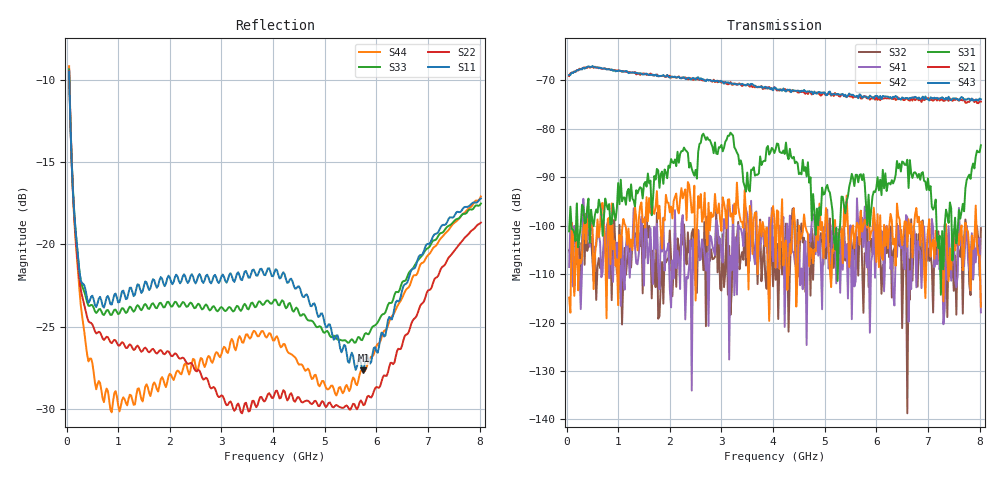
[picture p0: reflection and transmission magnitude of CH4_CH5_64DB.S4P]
!Agilent Technologies,E5071C,MY46316741,A.11.02
!Date: Mon Jun 01 11:46:35 2026
!Data & Calibration Information:
!1:CH4 INPUT 2:CH4 OUTPUT 3:CH5 INPUT 4:CH5 OUTPUT
!Freq	S11:SOLT4(ON)	S12:SOLT4(ON)	S13:SOLT4(ON)	S14:SOLT4(ON)
!	S21:SOLT4(ON)	S22:SOLT4(ON)	S23:SOLT4(ON)	S24:SOLT4(ON)
!	S31:SOLT4(ON)	S32:SOLT4(ON)	S33:SOLT4(ON)	S34:SOLT4(ON)
!	S41:SOLT4(ON)	S42:SOLT4(ON)	S43:SOLT4(ON)	S44:SOLT4(ON)
!PortZ  Port1:50+j0  Port2:50+j0  Port3:50+j0  Port4:50+j0
!Above PortZ is port z conversion or system Z0 setting when saving the data.
!When reading, reference impedance value at option line is always used.
# Hz S dB R 50
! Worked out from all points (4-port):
!   320 points, 50 MHz to 8.025 GHz, reference 50 ohm
!   strongest paths, dB at 50 MHz, 2.05 GHz, 4.05 GHz, 6.05 GHz, 8.025 GHz:
!     S43: -68.9, -69.2, -71.6, -73.6, -73.9
!     S21: -69.1, -69.3, -71.6, -73.4, -74.4
!     S31: -101.2, -86.9, -84.2, -92.7, -83.4
!     S42: -114.8, -98.5, -108.7, -108.6, -116.8
!     S41: -108.5, -107.2, -102.6, -102.5, -117.9
!     S32: -105.1, -114.6, -111.2, -107.1, -100.5
!   lowest |S11| = -27.7 dB at 5.75 GHz (marker M1), VSWR 1.09, Z = 47.1 - j2.84 ohm
!   |S11| at or under -10 dB: 53.85 MHz to end of sweep
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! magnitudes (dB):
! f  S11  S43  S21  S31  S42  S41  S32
! 50 MHz  -9.5  -68.9  -69.1  -101.2  -114.8  -108.5  -105.1
! 125 MHz  -16.9  -68.5  -68.3  -100.8  -101.9  -112.6  -107.4
! 275 MHz  -22.2  -67.7  -67.7  -99.9  -107.8  -117.2  -113.5
! 875 MHz  -23.7  -67.7  -67.8  -99.7  -95.4  -107.8  -115.4
! 4.05 GHz  -21.5  -71.6  -71.6  -84.2  -108.7  -102.6  -111.2
! 5.75 GHz  -27.7  -73.3  -73.3  -89.3  -100.1  -104.4  -118.0
! 8.025 GHz  -17.2  -73.9  -74.4  -83.4  -116.8  -117.9  -100.5
